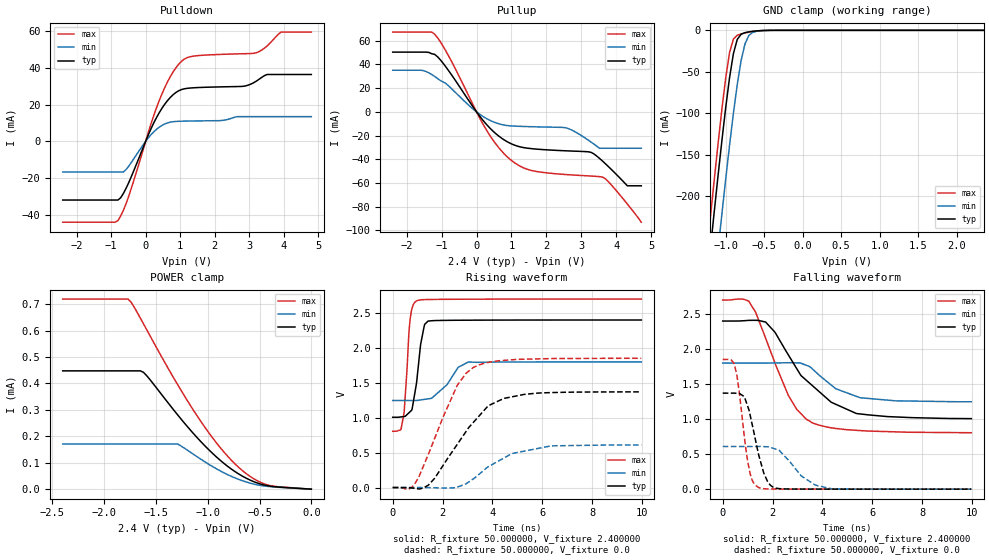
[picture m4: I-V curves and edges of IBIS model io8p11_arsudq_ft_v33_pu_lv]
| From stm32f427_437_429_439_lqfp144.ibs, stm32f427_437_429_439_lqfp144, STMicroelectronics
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|   Model io8p11_arsudq_ft_v33_pu_lv
[Model]  io8p11_arsudq_ft_v33_pu_lv
Model_type I/O
Polarity   Non-Inverting
Enable   Active-Low
Vinl =   0.720000V
Vinh =   1.680000V
Vmeas =  1.200000V
Cref =   30.000000pF
Rref =   100.000000M
Vref =   0.0V
C_comp   2.238700pF   2.180600pF   2.332300pF
[Temperature Range]   25.000000   0.125000k   -40.000000
[Pullup Reference]   2.400000V   1.800000V   2.700000V
[Pulldown Reference]   0.0V   0.0V   0.0V
[POWER Clamp Reference]   2.400000V   1.800000V   2.700000V
[GND Clamp Reference]   0.0V   0.0V   0.0V
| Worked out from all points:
|   slope of the pulldown table from 0 to 0.36 V, typ, clamps not added: 25 ohm
|   slope of the pullup table from 0 to 0.36 V, typ, clamps not added: 27.7 ohm
|   GND clamp passes 1 mA (typ) near -0.62 V on its own axis
|   rising waveform, R_fixture 50.000000, V_fixture 2.400000: 20-80 % time 303ps typ, 753ps min, 196ps max; typ from 1.01 V to 2.4 V
|   rising waveform, R_fixture 50.000000, V_fixture 0.0: 20-80 % time 1.7ns typ, 1.56ns min, 1.32ns max; typ from 0.001 V to 1.37 V
|   falling waveform, R_fixture 50.000000, V_fixture 2.400000: 20-80 % time 1.92ns typ, 1.43ns min, 1.35ns max; typ from 2.4 V to 1.01 V
|   falling waveform, R_fixture 50.000000, V_fixture 0.0: 20-80 % time 536ps typ, 998ps min, 390ps max; typ from 1.37 V to 0.001 V
[Pulldown]
|Voltage   I(typ)   I(min)   I(max)
-2.4V     -31.73mA   -16.51mA   -43.74mA
-800mV    -31.73mA   -16.51mA   -42.87mA
-480mV    -21.98mA   -13.17mA   -29.21mA
80mV      3.63mA     1.966mA    5.014mA
480mV     18.16mA    8.738mA    26.02mA
800mV     25.38mA    10.72mA    37.77mA
1.12V     28.53mA    11.02mA    44.6mA
2.8V      29.84mA    13.45mA    47.53mA
3.2V      32.59mA    13.45mA    48.03mA
3.52V     36.3mA     13.45mA    51.74mA
3.92V     36.3mA     13.45mA    59.27mA
4.8V      36.3mA     13.45mA    59.27mA
[Pullup]
|Voltage   I(typ)   I(min)   I(max)
-2.4V     50.37mA    35.09mA    67.27mA
-1.52V    50.37mA    34.75mA    67.27mA
-1.2V     48.49mA    29.88mA    65.45mA
-800mV    34.76mA    21.91mA    47.21mA
320mV     -11.75mA   -6.207mA   -17.08mA
1.04V     -27.53mA   -11.97mA   -41.91mA
1.6V      -31.13mA   -12.57mA   -49.63mA
2.56V     -32.88mA   -13.48mA   -52.9mA
3.28V     -34.18mA   -25.5mA    -54.17mA
3.6V      -41.3mA    -30.73mA   -54.97mA
4.32V     -62.41mA   -30.73mA   -77.79mA
4.72V     -62.41mA   -30.73mA   -93.1mA
[GND_clamp]
|Voltage   I(typ)   I(min)   I(max)
-2.4V     -1.424A    -1.508A    -1.394A
-1.25V    -311.2mA   -401.9mA   -273.3mA
-1.2V     -265.4mA   -356.1mA   -227.2mA
-1.15V    -220.4mA   -310.8mA   -181.9mA
-1.1V     -176.3mA   -266.2mA   -137.9mA
-1.05V    -133.8mA   -222.5mA   -95.87mA
-950mV    -57.3mA    -138.9mA   -26.98mA
-900mV    -28.27mA   -100.4mA   -10.59mA
-850mV    -11.01mA   -65.54mA   -5.958mA
-750mV    -2.834mA   -16.5mA    -3.178mA
-600mV    -750uA     -1.164mA   -738.3uA
2.35V     0A         0A         0A
[POWER_clamp]
|Voltage   I(typ)   I(min)   I(max)
-2.4V     447.7uA    170.8uA    719.3uA
-1.77V    447.7uA    170.8uA    719.3uA
-1.74V    447.7uA    170.8uA    707.6uA
-1.65V    447.7uA    170.8uA    647uA
-1.62V    442uA      170.8uA    625.5uA
-1.29V    280.9uA    170.8uA    395.1uA
-1.02V    161uA      101.5uA    230.1uA
-780mV    78.34uA    49.93uA    112.9uA
-600mV    36.03uA    23.94uA    50.74uA
-450mV    15.19uA    11.76uA    19.45uA
-330mV    8.429uA    7.427uA    9.749uA
0V        0A         0A         0A
[Ramp]
| variable   typ   min   max
dV/dt_r  0.82183/1.69891n   0.36910/1.63253n   1.11191/1.31895n
dV/dt_f  0.83106/1.91079n   0.33174/1.43600n   1.13538/1.35268n
R_load = 50.000000
[Rising Waveform]
R_fixture= 50.000000
V_fixture= 2.400000
V_fixture_min= 1.800000
V_fixture_max= 2.700000
|time   V(typ)   V(min)   V(max)
0s        1.007V     1.247V     806mV
320.3ps   1.012V     1.247V     827.7mV
440.4ps   1.017V     1.247V     1.04V
700.7ps   1.088V     1.247V     2.414V
961ps     1.514V     1.247V     2.673V
1.121ns   2.053V     1.255V     2.689V
1.281ns   2.338V     1.264V     2.692V
1.421ns   2.385V     1.271V     2.693V
3.043ns   2.397V     1.798V     2.698V
9.97ns    2.4V       1.8V       2.7V
[Rising Waveform]
R_fixture= 50.000000
V_fixture= 0.0
V_fixture_min= 0.0
V_fixture_max= 0.0
|time   V(typ)   V(min)   V(max)
0s        955.7uV    874.8uV    1.141mV
620.6ps   -1.541mV   858.3uV    -22.32mV
860.9ps   -10.25mV   901.5uV    40.49mV
1.441ns   39.2mV     82.9uV     488mV
2.583ns   616.3mV    5.559mV    1.46V
3.243ns   937.6mV    128.3mV    1.722V
3.844ns   1.174V     301.7mV    1.793V
5.245ns   1.333V     520.5mV    1.838V
6.366ns   1.361V     597.7mV    1.848V
9.97ns    1.371V     610.3mV    1.852V
[Falling Waveform]
R_fixture= 50.000000
V_fixture= 2.400000
V_fixture_min= 1.800000
V_fixture_max= 2.700000
|time   V(typ)   V(min)   V(max)
0s        2.4V       1.8V       2.7V
1.041ns   2.409V     1.8V       2.685V
1.321ns   2.41V      1.8V       2.524V
1.722ns   2.385V     1.8V       2.154V
2.643ns   1.911V     1.805V     1.332V
3.143ns   1.621V     1.797V     1.076V
3.604ns   1.476V     1.714V     945.9mV
4.545ns   1.21V      1.433V     866.3mV
5.506ns   1.074V     1.306V     837.3mV
9.97ns    1.007V     1.247V     806mV
[Falling Waveform]
R_fixture= 50.000000
V_fixture= 0.0
V_fixture_min= 0.0
V_fixture_max= 0.0
|time   V(typ)   V(min)   V(max)
0s        1.371V     610.3mV    1.852V
460.5ps   1.371V     610.2mV    1.789V
660.7ps   1.366V     610.1mV    1.392V
1.001ns   1.185V     609.9mV    398.1mV
1.441ns   490.7mV    610.7mV    25.04mV
1.802ns   107.9mV    605.7mV    4.671mV
2.202ns   11.05mV    562.3mV    2.86mV
3.143ns   2.463mV    191.5mV    2.026mV
4.384ns   1.637mV    4.533mV    1.627mV
9.97ns    955.7uV    874.8uV    1.141mV
